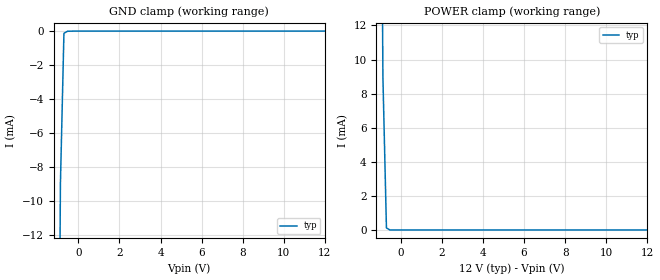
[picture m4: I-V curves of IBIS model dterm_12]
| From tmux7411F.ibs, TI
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| dterm_12
[Model]   dterm_12
Model_type   Terminator
|   typ   min   max
C_comp   4.014581e-12   NA   NA
[Voltage Range]   12   NA   NA
[Temperature Range]   27   NA   NA
[Power Clamp Reference]   12   NA   NA
[GND Clamp Reference]   0   NA   NA
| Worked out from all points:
|   GND clamp passes 1 mA (typ) near -0.72 V on its own axis
|   POWER clamp passes 1 mA (typ) near -0.72 V on its own axis
[GND Clamp]
|   Voltage   I(typ)   I(min)   I(max)
-5V       -1.049A    NA         NA
-1.051V   -41.26mA   NA         NA
-878.8mV  -8.99mA    NA         NA
-707.1mV  -128.8uA   NA         NA
-535.4mV  -9.633uA   NA         NA
12V       253.2pA    NA         NA
[POWER Clamp]
|   Voltage   I(typ)   I(min)   I(max)
-5V       1.049A     NA         NA
-1.05V    41.24mA    NA         NA
-878.8mV  8.978mA    NA         NA
-707.1mV  118.2uA    NA         NA
-535.4mV  575.6nA    NA         NA
12V       -282.7pA   NA         NA
